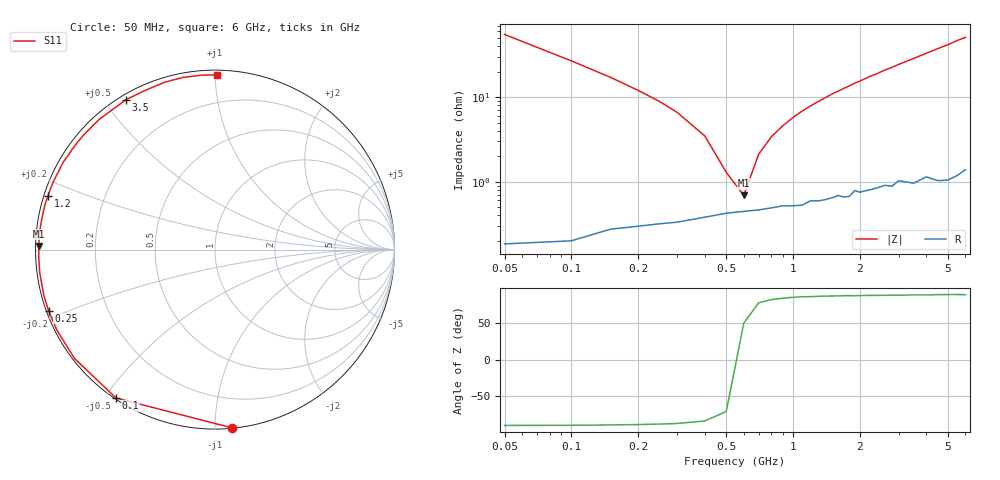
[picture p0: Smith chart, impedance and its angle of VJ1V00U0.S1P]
! Infineon Technologies  Discrete & RF Semiconductors
! BB 914
! Si Tuning Diode in SOT23
! VR = 1 V
! S-Parameters:  July  1999
# GHz  S  MA  R  50
!  f  S11
! GHz  MAG  ANG
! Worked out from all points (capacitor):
!   34 points, 50 MHz to 6 GHz, reference 50 ohm
!   read as one part to ground: C = 57.7 pF near 50 MHz
!   lowest |Z| = 687 mohm at 600 MHz (marker M1)
!   series resonance near 570 MHz, so ESL is about 1.4 nH
!   S11 on the Smith chart (normalised r, x): 50 MHz: 0.00, -1.10; 100 MHz: 0.00, -0.54; 250 MHz: 0.01, -0.18; 1.2 GHz: 0.01, +0.16; 3.5 GHz: 0.02, +0.57; 6 GHz: 0.03, +1.01
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0.05  0.9967 -84.7
0.1  0.9938 -123.7
0.15  0.9902 -142.2
0.2  0.9888 -153.0
0.25  0.9878 -159.9
0.3  0.987 -165.0
0.4  0.985 -172.1
0.5  0.9832 -177.2
0.6  0.9823 178.8
0.7  0.9817 175.3
0.8  0.9807 172.3
1  0.9797 167.0
1.2  0.9771 162.2
1.6  0.9743 153.6
1.8  0.9753 149.6
1.9  0.9715 147.5
2  0.9729 145.8
2.2  0.972 141.9
2.4  0.9709 138.5
2.6  0.9696 134.8
2.8  0.971 131.7
3  0.9673 128.2
3.5  0.9715 120.6
4  0.9687 113.3
4.5  0.9739 106.6
5  0.9756 100.6
5.5  0.975 94.2
6  0.9731 89.2
